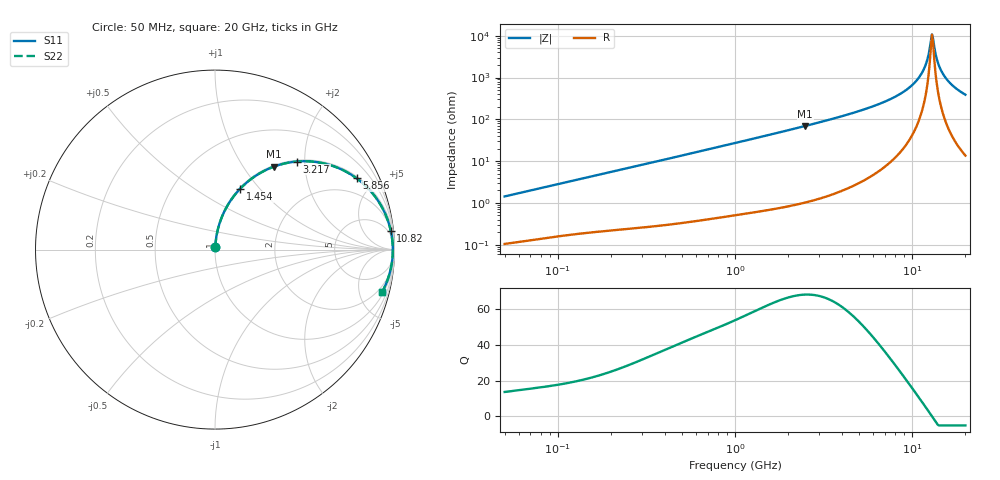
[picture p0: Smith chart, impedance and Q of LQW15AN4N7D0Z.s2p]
!Murata Part Number: LQW15AN4N7D0Z
!These Parameters are Measured in Series Mode Connection
!  o--[Z]--o
!Port1  Port2
!  o-------o
!Freq. Start=50[MHz] Stop=20[GHz], 401[Steps]
# Hz S RI R 50
!Freq.(Hz) S11(Real) S11(Imag) S21(Real) S21(Imag) S12(Real) S12(Imag) S22(Real) S22(Imag)
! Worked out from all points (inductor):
!   401 points, 50 MHz to 20 GHz, reference 50 ohm
!   read as one part in series: L = 4.5 nH near 51.52 MHz
!   highest Q = 67.9 at 2.494 GHz (marker M1), where L = 4.42 nH
!   self-resonance near 12.95 GHz
!   S11 on the Smith chart (normalised r, x): 50 MHz: 1.00, +0.03; 1.454 GHz: 1.01, +0.79; 3.217 GHz: 1.03, +1.83; 5.856 GHz: 1.09, +3.92; 10.82 GHz: 3, +19; 20 GHz: 1.27, -7.76
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5e7  0.00124 0.0142  0.9988 -0.0142  0.9988 -0.0142  0.00124 0.0142
1.364002e8  0.00327 0.0375  0.9967 -0.0375  0.9967 -0.0375  0.00327 0.0375
3.721004e8  0.0129 0.0995  0.9871 -0.0995  0.9871 -0.0995  0.0129 0.0995
1e9  0.0722 0.2496  0.9278 -0.2496  0.9278 -0.2496  0.0722 0.2496
1.454215e9  0.1389 0.3377  0.8611 -0.3377  0.8611 -0.3377  0.1389 0.3377
2.493527e9  0.3263 0.4616  0.6737 -0.4616  0.6737 -0.4616  0.3263 0.4616
2.728004e9  0.3697 0.4754  0.6303 -0.4754  0.6303 -0.4754  0.3697 0.4754
3.216634e9  0.4567 0.4906  0.5433 -0.4906  0.5433 -0.4906  0.4567 0.4906
5.856089e9  0.7888 0.3974  0.2112 -0.3974  0.2112 -0.3974  0.7888 0.3974
7.442007e9  0.8902 0.2978  0.1098 -0.2978  0.1098 -0.2978  0.8902 0.2978
9.316812e9  0.9548 0.1843  0.0452 -0.1843  0.0452 -0.1843  0.9548 0.1843
1.082228e10  0.9799 0.1024  0.0201 -0.1024  0.0201 -0.1024  0.9799 0.1024
1.183995e10  0.988 0.052  0.012 -0.052  0.012 -0.052  0.988 0.052
1.220001e10  0.9895 0.0351  0.0105 -0.0351  0.0105 -0.0351  0.9895 0.0351
1.276073e10  0.9907 0.00964  0.00929 -0.00964  0.00929 -0.00964  0.9907 0.00964
1.295331e10  0.9908 0.00115  0.00918 -0.00115  0.00918 -0.00115  0.9908 0.00115
1.334722e10  0.9906 -0.0158  0.00941 0.0158  0.00941 0.0158  0.9906 -0.0158
1.375312e10  0.9898 -0.0328  0.0102 0.0328  0.0102 0.0328  0.9898 -0.0328
1.417136e10  0.9884 -0.0497  0.0116 0.0497  0.0116 0.0497  0.9884 -0.0497
1.504638e10  0.9839 -0.0835  0.0161 0.0835  0.0161 0.0835  0.9839 -0.0835
1.696185e10  0.9678 -0.15  0.0322 0.15  0.0322 0.15  0.9678 -0.15
2e10  0.9305 -0.2375  0.0695 0.2375  0.0695 0.2375  0.9305 -0.2375
